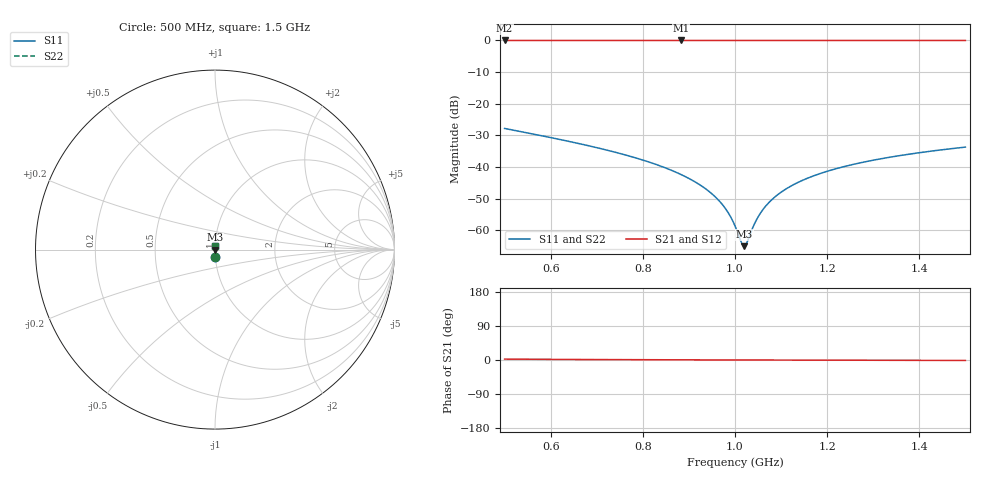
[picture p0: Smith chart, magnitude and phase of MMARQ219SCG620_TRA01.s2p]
! MMARQ219SCG620_TRA01  S-PARAMETER MODEL  ( General Type )
! Model Generated by TAIYO YUDEN Corporation (http://www.ty-top.com)
! Version 1.0
! TAIYO YUDEN Control No. 150609
! Copyright(c) 2015 TAIYO YUDEN CO.,LTD. All Rights Reserved.
! Product Description (link to TY-COMPAS)
! https://ds.yuden.co.jp/TYCOMPAS/or/detail?pn=MMARQ219SCG620JTRA01&u=M
! Products Name : Multilayer Ceramic Capacitors
! Characteristics :
!  Capacitance : 62 pF , Rated Voltage : 250V , TCC : CG / C0G
!  Case Size : 2.0 x 1.25 / 0.079 x 0.049 [mm/inch] , Thickness : 0.85 / 0.033 [mm/inch]
!  (Conditions: Temperature = 25 degC , DC Bias Current/Voltage = 0A / 0V)
! External Node Assignments :
!  1  o---| |---o  2
! GND o---------o GND
! Frequency Range : 500MHz  -  1.5GHz  [ 401 STEP ]
# MHz S RI R 50
! Freq[MHz].  S11 Real  S11 Imag  S21 Real  S21 Imag  S12 Real  S12 Imag  S22 Real  S22 Imag
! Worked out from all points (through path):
!   401 points, 500 MHz to 1.5 GHz, reference 50 ohm
!   highest |S21| = 0.00 dB at 882.5 MHz (marker M1); lowest = 0.0 dB at 500 MHz (marker M2)
!   lowest |S11| = -65.0 dB at 1.02 GHz (marker M3), VSWR 1.00, Z = 50.1 - j1.76e-05 ohm
!   |S11| at or under -10 dB: start of sweep to end of sweep
!   |S22| runs from -65.0 to -27.8 dB; largest |S21 - S12| = 0
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500  0.00199 -0.0406  0.998 0.0406  0.998 0.0406  0.00199 -0.0406
667.5  0.000927 -0.0229  0.9991 0.0229  0.9991 0.0229  0.000927 -0.0229
762.5  0.000682 -0.0155  0.9993 0.0155  0.9993 0.0155  0.000682 -0.0155
835  0.000587 -0.0106  0.9994 0.0106  0.9994 0.0106  0.000587 -0.0106
882.5  0.000555 -0.00761  0.9994 0.00761  0.9994 0.00761  0.000555 -0.00761
925  0.000543 -0.00513  0.9995 0.00513  0.9995 0.00513  0.000543 -0.00513
957.5  0.000543 -0.00331  0.9995 0.00331  0.9995 0.00331  0.000543 -0.00331
982.5  0.000547 -0.00196  0.9995 0.00196  0.9995 0.00196  0.000547 -0.00196
1000  0.000553 -0.00104  0.9994 0.00104  0.9994 0.00104  0.000553 -0.00104
1012.5  0.000558 -0.000386  0.9994 0.000386  0.9994 0.000386  0.000558 -0.000386
1020  0.000561 -1.76e-07  0.9994 1.76e-07  0.9994 1.76e-07  0.000561 -1.76e-07
1027.5  0.000565 0.000383  0.9994 -0.000383  0.9994 -0.000383  0.000565 0.000383
1040  0.000571 0.00102  0.9994 -0.00102  0.9994 -0.00102  0.000571 0.00102
1050  0.000577 0.00152  0.9994 -0.00152  0.9994 -0.00152  0.000577 0.00152
1062.5  0.000585 0.00213  0.9994 -0.00213  0.9994 -0.00213  0.000585 0.00213
1075  0.000594 0.00275  0.9994 -0.00275  0.9994 -0.00275  0.000594 0.00275
1092.5  0.000608 0.00359  0.9994 -0.00359  0.9994 -0.00359  0.000608 0.00359
1115  0.000627 0.00466  0.9994 -0.00466  0.9994 -0.00466  0.000627 0.00466
1167.5  0.00068 0.00708  0.9993 -0.00708  0.9993 -0.00708  0.00068 0.00708
1240  0.00077 0.0103  0.9992 -0.0103  0.9992 -0.0103  0.00077 0.0103
1335  0.00091 0.0142  0.9991 -0.0142  0.9991 -0.0142  0.00091 0.0142
1500  0.00121 0.0206  0.9988 -0.0206  0.9988 -0.0206  0.00121 0.0206
